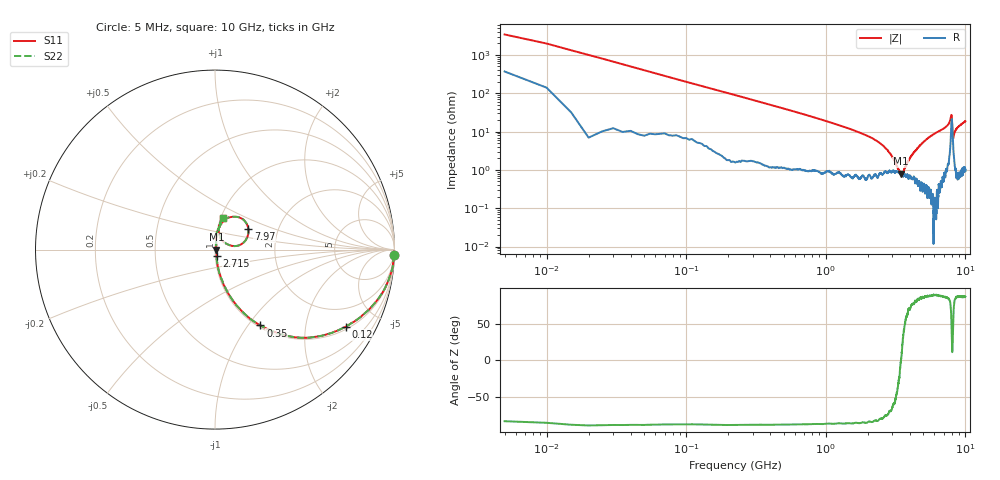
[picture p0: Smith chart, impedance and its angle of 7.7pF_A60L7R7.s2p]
! Amotech Co.,Ltd.
! http://www.amotech.co.kr/
! Part Number: A60L7R7
! These Parameters are Measured in Series Mode Connection
! Operation Temp=25[degC], DC Bias Voltage=0[V]
! Freq. Start=5[MHz] Stop=10[GHz], 2000[Steps]
! Date: Monday, July 14, 2020, 09:55:29
# GHZ S RI R 50.000000
!Freq.(Hz) S11(Real) S11(Imag) S21(Real) S21(Imag) S12(Real) S12(Imag) S22(Real) S22(Imag)
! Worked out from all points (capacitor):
!   2000 points, 5 MHz to 10 GHz, reference 50 ohm
!   read as one part in series: C = 7.99 pF near 55 MHz
!   lowest |Z| = 797 mohm at 3.445 GHz (marker M1)
!   series resonance near 3.455 GHz, so ESL is about 270 pH
!   S11 on the Smith chart (normalised r, x): 5 MHz: 8, -68; 120 MHz: 1.10, -3.33; 350 MHz: 1.03, -1.15; 2.715 GHz: 1.02, -0.07; 7.97 GHz: 1.41, +0.34; 10 GHz: 1.02, +0.37
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0.005  0.996 -0.0288  0.00398 0.0288  0.00398 0.0288  0.996 -0.0288
0.07  0.8826 -0.3065  0.1174 0.3065  0.1174 0.3065  0.8826 -0.3065
0.12  0.7283 -0.4296  0.2717 0.4296  0.2717 0.4296  0.7283 -0.4296
0.205  0.4922 -0.4909  0.5078 0.4909  0.5078 0.4909  0.4922 -0.4909
0.35  0.2527 -0.4227  0.7473 0.4227  0.7473 0.4227  0.2527 -0.4227
0.74  0.0727 -0.2428  0.9273 0.2428  0.9273 0.2428  0.0727 -0.2428
1.675  0.0166 -0.0973  0.9834 0.0973  0.9834 0.0973  0.0166 -0.0973
2.715  0.00973 -0.0335  0.9903 0.0335  0.9903 0.0335  0.00973 -0.0335
3.34  0.00896 -0.00423  0.991 0.00423  0.991 0.00423  0.00896 -0.00423
3.445  0.00789 -0.0005  0.9921 0.0005  0.9921 0.0005  0.00789 -0.0005
3.58  0.00742 0.00435  0.9926 -0.00435  0.9926 -0.00435  0.00742 0.00435
3.845  0.00733 0.0143  0.9927 -0.0143  0.9927 -0.0143  0.00733 0.0143
4.23  0.00666 0.0263  0.9933 -0.0263  0.9933 -0.0263  0.00666 0.0263
5.005  0.00649 0.0524  0.9935 -0.0524  0.9935 -0.0524  0.00649 0.0524
6.67  0.0166 0.107  0.9834 -0.107  0.9834 -0.107  0.0166 0.107
7.645  0.0446 0.1558  0.9554 -0.1558  0.9554 -0.1558  0.0446 0.1558
7.875  0.1149 0.1828  0.8851 -0.1828  0.8851 -0.1828  0.1149 0.1828
7.97  0.1857 0.1141  0.8143 -0.1141  0.8143 -0.1141  0.1857 0.1141
8.145  0.0508 0.0406  0.9492 -0.0406  0.9492 -0.0406  0.0508 0.0406
8.335  0.0231 0.0858  0.9769 -0.0858  0.9769 -0.0858  0.0231 0.0858
8.71  0.0223 0.1199  0.9777 -0.1199  0.9777 -0.1199  0.0223 0.1199
10  0.0424 0.1774  0.9576 -0.1774  0.9576 -0.1774  0.0424 0.1774
